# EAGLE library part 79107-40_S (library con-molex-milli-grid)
RECEPTACAL
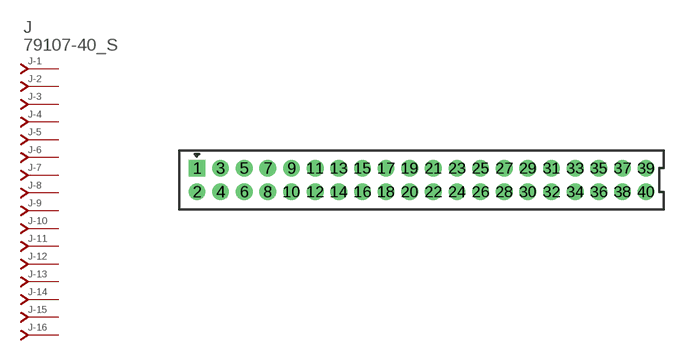
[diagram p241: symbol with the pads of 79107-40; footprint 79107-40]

Designator prefix J; gates -1=J-NV -2=J-N -3=J-N -4=J-N -5=J-N -6=J-N -7=J-N -8=J-N -9=J-N -10=J-N -11=J-N -12=J-N -13=J-N -14=J-N -15=J-N -16=J-N -17=J-N -18=J-N -19=J-N -20=J-N -21=J-N -22=J-N -23=J-N -24=J-N -25=J-N -26=J-N -27=J-N -28=J-N -29=J-N -30=J-N -31=J-N -32=J-N -33=J-N -34=J-N -35=J-N -36=J-N -37=J-N -38=J-N -39=J-N -40=J-N

## 79107-40_S  [79107-40]
1  -1:J  pas
2  -2:J  pas
3  -3:J  pas
4  -4:J  pas
5  -5:J  pas
6  -6:J  pas
7  -7:J  pas
8  -8:J  pas
9  -9:J  pas
10  -10:J  pas
11  -11:J  pas
12  -12:J  pas
13  -13:J  pas
14  -14:J  pas
15  -15:J  pas
16  -16:J  pas
17  -17:J  pas
18  -18:J  pas
19  -19:J  pas
20  -20:J  pas
21  -21:J  pas
22  -22:J  pas
23  -23:J  pas
24  -24:J  pas
25  -25:J  pas
26  -26:J  pas
27  -27:J  pas
28  -28:J  pas
29  -29:J  pas
30  -30:J  pas
31  -31:J  pas
32  -32:J  pas
33  -33:J  pas
34  -34:J  pas
35  -35:J  pas
36  -36:J  pas
37  -37:J  pas
38  -38:J  pas
39  -39:J  pas
40  -40:J  pas

## Footprint 79107-40 (pad centres in mm)
RECEPTACAL Dual Row, Vertical, Through-Hole
drill 0.914 square: 1 -19,1
drill 0.914: 2 -19,-1; 3 -17,1; 4 -17,-1; 5 -15,1; 6 -15,-1; 7 -13,1; 8 -13,-1; 9 -11,1; 10 -11,-1; 11 -9,1; 12 -9,-1; 13 -7,1; 14 -7,-1; 15 -5,1; 16 -5,-1; 17 -3,1; 18 -3,-1; 19 -1,1; 20 -1,-1; 21 1,1; 22 1,-1; 23 3,1; 24 3,-1; 25 5,1; 26 5,-1; 27 7,1; 28 7,-1; 29 9,1; 30 9,-1; 31 11,1; 32 11,-1; 33 13,1; 34 13,-1; 35 15,1; 36 15,-1; 37 17,1; 38 17,-1; 39 19,1; 40 19,-1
